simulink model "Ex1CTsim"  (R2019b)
settings: Solver=FixedStepAuto  StartTime=0.0  StopTime=25.0  FixedStep=h/100  RelTol=1e-3
libraries: cstblocks x3

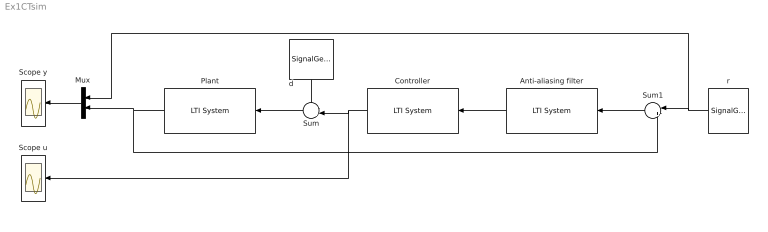
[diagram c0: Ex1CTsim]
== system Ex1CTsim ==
  Anti-aliasing filter : cstblocks/LTI System  sys=Fpsi  IC=[]
  Controller : cstblocks/LTI System  sys=Cdtpr  IC=[]
  Mux : Mux  Inputs=2
  Plant : cstblocks/LTI System  sys=Pc  IC=[]
  Scope u : Scope
  Scope y : Scope
  Sum : Sum  Inputs=++|
  Sum1 : Sum  Inputs=|+-
  d : SignalGenerator  WaveForm=square  Amplitude=.5  Frequency=pi/12  Units=rad/sec
  r : SignalGenerator  Amplitude=0  Frequency=pi/15  Units=rad/sec
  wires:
  Anti-aliasing filter/1 -> Controller/1
  Sum/1 -> Plant/1
  d/1 -> Sum/1
  Sum1/1 -> Anti-aliasing filter/1
  Plant/1 -> Mux/2, Sum1/2
  Controller/1 -> Scope u/1, Sum/2
  r/1 -> Mux/1, Sum1/1
  Mux/1 -> Scope y/1
